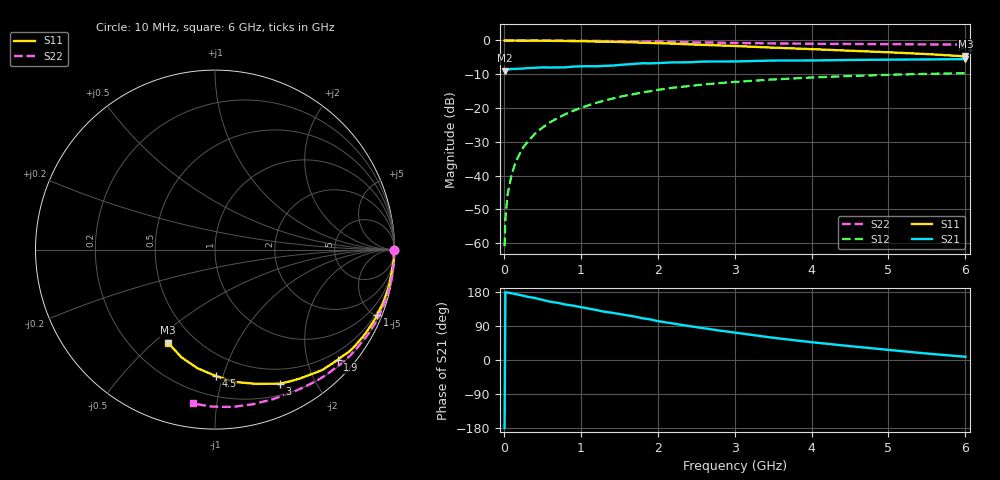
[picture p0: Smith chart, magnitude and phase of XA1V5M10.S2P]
! SIEMENS Discrete & RF Semiconductors
! BFY180
! Si NPN RF Bipolar Junction Transistor in MICRO-X
! VCE = 1.5 V  IC = 0.1 mA
! Common Emitter S-Parameters:  May  1997
# GHz  S  MA  R  50
!  f  S11  S21  S12  S22
! GHz  MAG  ANG  MAG  ANG  MAG  ANG  MAG  ANG
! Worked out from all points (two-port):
!   36 points, 10 MHz to 6 GHz, reference 50 ohm
!   highest |S21| = -5.53 dB at 6 GHz (marker M1); lowest = -9.0 dB at 10 MHz (marker M2)
!   |S21| within 3 dB of the highest: 75.17 MHz to end of sweep
!   lowest |S11| = -4.7 dB at 6 GHz (marker M3), VSWR 3.78, Z = 17.7 - j27.8 ohm
!   |S11| at or under -10 dB: nowhere
!   |S22| runs from -1.2 to 0.0 dB; largest |S21 - S12| = 0.39
!   S11 on the Smith chart (normalised r, x): 10 MHz: open; 1 GHz: 0.34, -5.12; 1.9 GHz: 0.32, -2.57; 3 GHz: 0.32, -1.54; 4.5 GHz: 0.34, -0.95; 6 GHz: 0.35, -0.56
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0.01  0.9962 0.0  0.355 -179.8  0.0009 99.6  0.9993 -0.1
0.02  0.9999 -0.4  0.364 178.9  0.0023 92.1  0.9999 -0.4
0.05  0.9947 -1.0  0.37 177.7  0.0054 86.5  0.9991 -0.9
0.1  0.9966 -2.1  0.379 176.2  0.0102 88.7  0.9975 -1.9
0.15  0.9983 -3.4  0.379 173.9  0.0155 87.4  0.9999 -2.9
0.25  0.9941 -5.5  0.384 169.8  0.0259 84.7  0.9999 -4.8
0.4  0.9914 -8.7  0.393 163.7  0.0412 82.3  0.9982 -7.7
0.6  0.9879 -13.2  0.398 153.9  0.0613 78.1  0.9962 -11.6
0.8  0.9827 -17.7  0.4 146.4  0.0809 73.8  0.9928 -15.5
1  0.9754 -22.0  0.414 139.5  0.1003 69.4  0.9888 -19.4
1.1  0.97 -24.2  0.416 135.8  0.1093 67.5  0.9859 -21.2
1.5  0.9493 -33.1  0.433 121.5  0.1459 59.1  0.9746 -28.8
1.8  0.9249 -40.0  0.46 110.2  0.1697 53.5  0.9633 -34.4
1.9  0.9193 -42.0  0.458 107.4  0.177 51.4  0.9596 -36.1
2.2  0.8982 -48.4  0.474 96.3  0.1996 45.6  0.9508 -41.6
2.6  0.8599 -56.6  0.487 83.8  0.2231 38.5  0.9339 -48.1
3  0.8288 -64.3  0.489 72.4  0.2429 31.6  0.9182 -54.6
3.5  0.7825 -73.0  0.504 58.7  0.2648 24.3  0.9049 -61.8
4  0.7447 -81.7  0.506 47.0  0.2827 17.1  0.8933 -69.1
4.5  0.7045 -89.6  0.514 36.6  0.2974 10.3  0.8869 -76.4
5.5  0.6288 -107.2  0.524 17.0  0.3202 -2.8  0.875 -91.1
6  0.5812 -117.0  0.529 8.5  0.3272 -9.5  0.8663 -98.3
